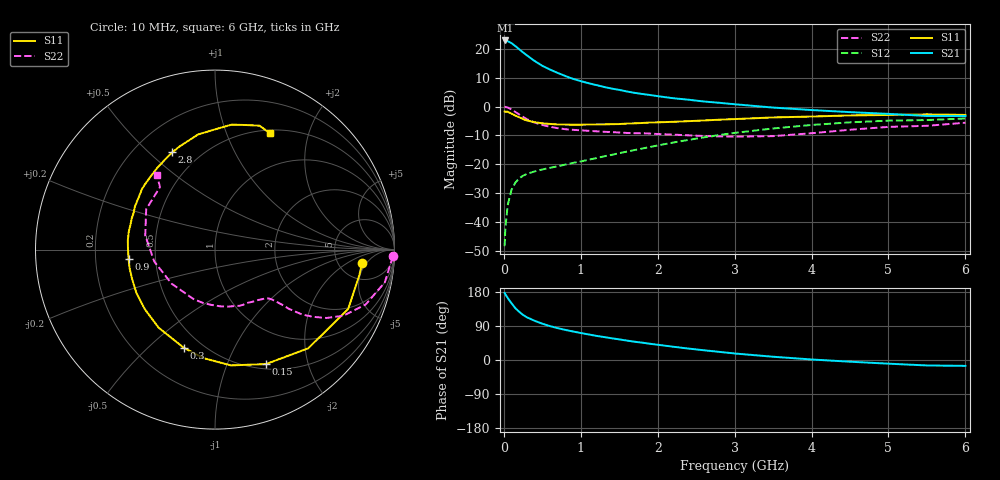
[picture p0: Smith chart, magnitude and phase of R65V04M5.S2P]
! SIEMENS Small Signal Semiconductors
! BFR193
! Si NPN RF Bipolar Junction Transistor in SOT23
! VCE = 5 V  IC = 4.5 mA
! Common Emitter S-Parameters:  May  1996
# GHz  S  MA  R  50
!  f  S11  S21  S12  S22
! GHz  MAG  ANG  MAG  ANG  MAG  ANG  MAG  ANG
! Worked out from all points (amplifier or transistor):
!   36 points, 10 MHz to 6 GHz, reference 50 ohm
!   highest |S21| = 22.9 dB at 20 MHz (marker M1)
!   |S21| within 3 dB of that: start of sweep to 197.7 MHz
!   unconditionally stable (mu >= 1): 938.4 MHz to 1.987 GHz
!   at 250 MHz: K = 0.40, MSG = 21.4 dB, |S12| = -24.0 dB
!   at 1.4 GHz: K = 1.07, MAG = 9.9 dB, |S12| = -16.7 dB
!   at 6 GHz: K = 0.96, MSG = 0.4 dB, |S12| = -4.1 dB
!   S11 on the Smith chart (normalised r, x): 10 MHz: 8.54, -3.89; 150 MHz: 0.56, -1.39; 300 MHz: 0.40, -0.65; 900 MHz: 0.35, -0.05; 2.8 GHz: 0.36, +0.59; 6 GHz: 0.54, +1.44
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0.01  0.8235 -5.1  13.98 176.9  0.0038 87.1  0.9926 -2.2
0.02  0.8168 -10.0  14.01 173.2  0.0078 85.5  0.9821 -4.4
0.05  0.8123 -24.1  13.62 163.9  0.0195 77.6  0.9636 -10.9
0.1  0.7566 -46.6  12.57 149.5  0.0361 68.0  0.8937 -20.0
0.15  0.6982 -66.0  11.19 136.7  0.0482 59.5  0.8052 -27.2
0.2  0.6512 -82.2  9.86 127.1  0.0571 54.0  0.729 -31.5
0.25  0.6076 -96.3  8.69 119.0  0.0633 50.2  0.6612 -34.5
0.3  0.5736 -107.7  7.714 112.6  0.0681 48.3  0.6045 -36.7
0.4  0.5365 -125.9  6.174 103.5  0.0751 46.2  0.5282 -38.7
0.5  0.5129 -139.6  5.092 95.8  0.0813 45.9  0.4796 -39.5
0.6  0.5002 -151.1  4.384 89.4  0.0866 47.1  0.4461 -40.4
0.7  0.4902 -160.1  3.833 84.1  0.0923 48.4  0.4222 -41.2
0.9  0.4844 -174.0  3.024 75.2  0.1056 51.3  0.3951 -43.4
1.1  0.4885 173.8  2.545 67.5  0.1195 54.4  0.3799 -46.8
1.3  0.491 163.8  2.193 60.6  0.1369 56.8  0.3655 -50.6
1.6  0.5069 151.6  1.827 51.2  0.166 58.9  0.3488 -57.9
2.2  0.544 130.8  1.396 35.1  0.2379 58.2  0.3265 -76.7
2.8  0.5921 113.7  1.163 21.5  0.321 52.4  0.3044 -103.0
3.5  0.6482 98.4  0.961 8.6  0.4171 41.7  0.3074 -141.8
4.5  0.7024 82.4  0.801 -4.5  0.533 24.7  0.3965 168.5
5.5  0.7336 70.2  0.687 -14.4  0.5838 7.1  0.4641 131.3
6  0.7167 64.6  0.686 -15.5  0.6214 2.1  0.5247 128.0
